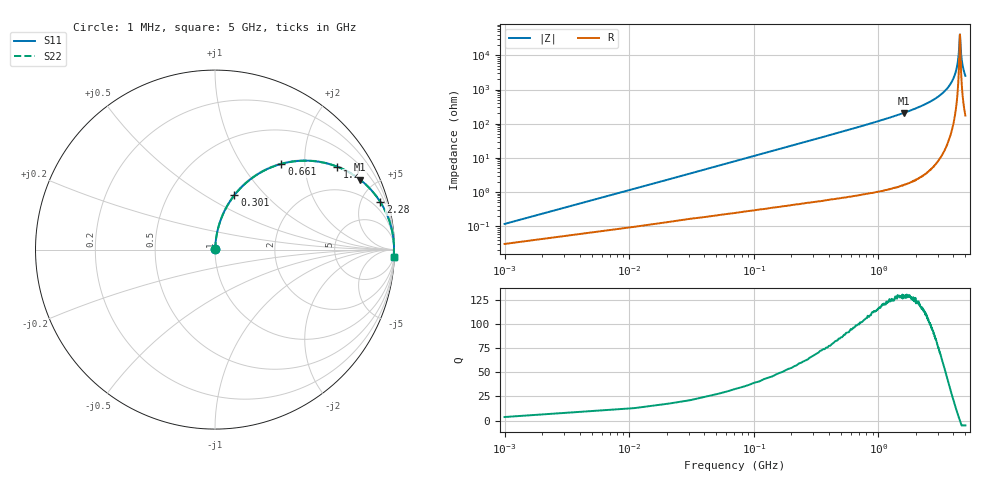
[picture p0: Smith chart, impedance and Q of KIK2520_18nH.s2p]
!version-2
!date-01.2022
!Series
# MHz S RI R 50
!Freq ReS11 ImS11 ReS21 ImS21 ReS12 ImS12 ReS22 ImS22
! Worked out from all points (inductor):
!   501 points, 1 MHz to 5 GHz, reference 50 ohm
!   read as one part in series: L = 18 nH near 21 MHz
!   highest Q = 129 at 1.6 GHz (marker M1), where L = 20.6 nH
!   self-resonance near 4.51 GHz
!   S11 on the Smith chart (normalised r, x): 1 MHz: 1.00, +0.00; 301 MHz: 1.01, +0.68; 661 MHz: 1.02, +1.53; 1.2 GHz: 1.02, +2.92; 2.28 GHz: 1.06, +6.92; 5 GHz: 5, -50
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1  0.000311 0.00113  0.9997 -0.00113  0.9997 -0.00113  0.000311 0.00113
31  0.00285 0.0349  0.9971 -0.0349  0.9971 -0.0349  0.00285 0.0349
51  0.00538 0.0573  0.9946 -0.0573  0.9946 -0.0573  0.00538 0.0573
71  0.00882 0.0794  0.9912 -0.0794  0.9912 -0.0794  0.00882 0.0794
161  0.0355 0.1752  0.9645 -0.1752  0.9645 -0.1752  0.0355 0.1752
301  0.1083 0.3034  0.8917 -0.3034  0.8917 -0.3034  0.1083 0.3034
661  0.3698 0.4777  0.6302 -0.4777  0.6302 -0.4777  0.3698 0.4777
841  0.4927 0.4953  0.5073 -0.4953  0.5073 -0.4953  0.4927 0.4953
1200  0.6798 0.4625  0.3202 -0.4625  0.3202 -0.4625  0.6798 0.4625
1600  0.809 0.3892  0.191 -0.3892  0.191 -0.3892  0.809 0.3892
1670  0.8254 0.3757  0.1746 -0.3757  0.1746 -0.3757  0.8254 0.3757
2280  0.921 0.2654  0.079 -0.2654  0.079 -0.2654  0.921 0.2654
2510  0.9421 0.2288  0.0579 -0.2288  0.0579 -0.2288  0.9421 0.2288
3340  0.9838 0.1179  0.0162 -0.1179  0.0162 -0.1179  0.9838 0.1179
3840  0.9938 0.0634  0.00622 -0.0634  0.00622 -0.0634  0.9938 0.0634
4170  0.9967 0.0313  0.00327 -0.0313  0.00327 -0.0313  0.9967 0.0313
4380  0.9975 0.0122  0.00252 -0.0122  0.00252 -0.0122  0.9975 0.0122
4520  0.9976 -9.03e-05  0.00244 9.03e-05  0.00244 9.03e-05  0.9976 -9.03e-05
4610  0.9975 -0.00776  0.00255 0.00776  0.00255 0.00776  0.9975 -0.00776
4690  0.9973 -0.0145  0.00274 0.0145  0.00274 0.0145  0.9973 -0.0145
4820  0.9968 -0.0251  0.00324 0.0251  0.00324 0.0251  0.9968 -0.0251
5000  0.9957 -0.0393  0.00426 0.0393  0.00426 0.0393  0.9957 -0.0393
